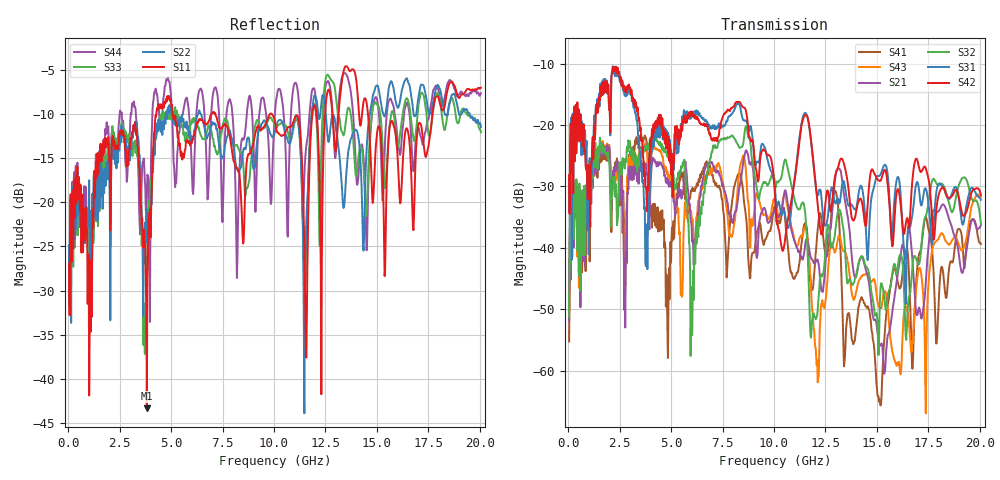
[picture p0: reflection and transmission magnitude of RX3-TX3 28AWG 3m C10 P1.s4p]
! FILE: O:\PROJECTS\SI-2007-05-003 3m Eyemax Qual\XT\FD\RX3-TX3 28AWG 3m C10 P1.s4p
# MHZ S RI R 50.00
! FREQ  S11  S12  S13  S14
!  S21  S22  S23  S24
!  S31  S32  S33  S34
!  S41  S42  S43  S44
!  REAL  IMAG  REAL  IMAG  REAL  IMAG  REAL  IMAG
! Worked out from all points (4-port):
!   801 points, 50 MHz to 20.05 GHz, reference 50 ohm
!   strongest paths, dB at 50 MHz, 5.05 GHz, 10.05 GHz, 15.05 GHz, 20.05 GHz:
!     S42: -28.1, -25.8, -31.5, -28.9, -31.5
!     S31: -28.8, -29.0, -30.1, -28.3, -32.2
!     S32: -51.3, -26.3, -29.4, -54.3, -36.0
!     S21: -51.8, -30.3, -33.9, -54.4, -36.3
!     S43: -51.3, -27.8, -32.1, -49.2, -31.8
!     S41: -55.3, -36.7, -33.4, -64.2, -39.4
!   lowest |S11| = -43.3 dB at 3.825 GHz (marker M1), VSWR 1.01, Z = 49.7 + j0.629 ohm
!   |S11| at or under -10 dB: start of sweep to 4.287 GHz; 7.156 GHz to 9.809 GHz (2.653 GHz wide, 31.3 % of centre); 14.56 GHz to 17.7 GHz (3.131 GHz wide, 19.4 % of centre)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
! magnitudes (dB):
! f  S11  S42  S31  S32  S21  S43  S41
! 50 MHz  -27.0  -28.1  -28.8  -51.3  -51.8  -51.3  -55.3
! 2.325 GHz  -13.6  -10.5  -10.7  -29.6  -27.2  -27.5  -27.1
! 3.825 GHz  -43.3  -34.0  -36.2  -23.3  -28.0  -24.0  -22.9
! 4.85 GHz  -8.3  -24.5  -21.3  -25.0  -28.9  -28.3  -58.0
! 12.97 GHz  -14.1  -28.3  -32.7  -37.4  -28.7  -40.6  -30.7
! 15.12 GHz  -11.6  -29.1  -28.3  -51.2  -55.8  -49.7  -64.7
! 20.05 GHz  -7.0  -31.5  -32.2  -36.0  -36.3  -31.8  -39.4
